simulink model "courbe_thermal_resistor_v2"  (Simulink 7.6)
settings: Solver=ode15s  StartTime=0.0  StopTime=500  RelTol=1e-3
InitFcn:
  | Vcc=12;
  | R=1e3;
  | 
  | T0=25+273.15;
  | R0=1;
  | alpha=5e-5;
StopFcn:
  | close all
  | load Te_appliquee_Tcalculee.mat
  | plot(x(1,:),x(2,:))
  | hold on
  | plot (x(1,:),x(3,:))
  | title('Température appliquée et mesurée')
  | xlabel('temps')
  | grid
undefined symbols (not defined in the file or in its folder): sigbuilder_block
libraries: fl_lib x17, nesl_utility x3, elec_lib x2

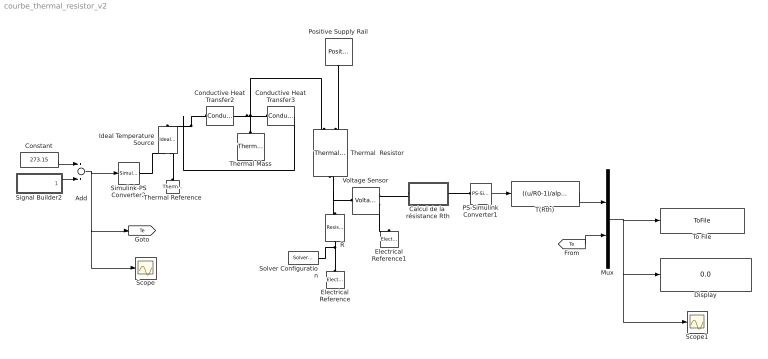
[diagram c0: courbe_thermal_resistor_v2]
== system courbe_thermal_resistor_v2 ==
  Add : Sum  Inputs=2
  Calcul de la  résistance Rth : Subsystem
  Conductive Heat Transfer2 : fl_lib/Thermal/Thermal Elements/Conductive Heat Transfer  DialogController=NetworkEngine.DynNeDlgSource  SystemSampleTime=-1  area=0.04 m^2  thickness=0.1 m  th_cond=46 W/(m*K)  Q_Log=off  T_Log=off  LocalVarNames=|Q|T  LocalVarDescs=|Q|T  LocalVarLogging=[0 0]
  Conductive Heat Transfer3 : fl_lib/Thermal/Thermal Elements/Conductive Heat Transfer  DialogController=NetworkEngine.DynNeDlgSource  SystemSampleTime=-1  area=0.04 m^2  thickness=0.1 m  th_cond=46 W/(m*K)  Q_Log=off  T_Log=off  LocalVarNames=|Q|T  LocalVarDescs=|Q|T  LocalVarLogging=[0 0]
  Constant : Constant  Value=273.15
  Display : Display
  Electrical Reference : fl_lib/Electrical/Electrical Elements/Electrical Reference  DialogController=NetworkEngine.DynNeDlgSource  SystemSampleTime=-1  i_Log=off  LocalVarNames=|i  LocalVarDescs=|i  LocalVarLogging=[]
  Electrical Reference1 : fl_lib/Electrical/Electrical Elements/Electrical Reference  DialogController=NetworkEngine.DynNeDlgSource  SystemSampleTime=-1  i_Log=off  LocalVarNames=|i  LocalVarDescs=|i  LocalVarLogging=[]
  Ideal Temperature Source : fl_lib/Thermal/Thermal Sources/Ideal Temperature Source  DialogController=NetworkEngine.DynNeDlgSource  SystemSampleTime=-1  Q_Log=off  T_Log=off  LocalVarNames=|Q|T  LocalVarDescs=|Q|T  LocalVarLogging=[0 0]
  Mux : Mux  Inputs=2
  PS-Simulink Converter1 : nesl_utility/PS-Simulink Converter  DialogController=NetworkEngine.DynNeUtilDlgSource  SystemSampleTime=-1  PhysicalDomain=network_engine_domain  LeftPortType=input  RightPortType=output  SubClassName=ps_output  Unit=V  AffineConversion=off
  Positive Supply Rail : elec_lib/Sources/Positive Supply Rail  DialogController=NetworkEngine.DynNeDlgSource  SystemSampleTime=-1  v0=Vcc V  current_Log=off  voltage_Log=off  power_Log=off  LocalVarNames=|current|voltage|power  LocalVarDescs=|Current (A)|Voltage (V)|Power (W)  LocalVarLogging=[0 0 0]
  R : fl_lib/Electrical/Electrical Elements/Resistor  DialogController=NetworkEngine.DynNeDlgSource  SystemSampleTime=-1  R=R Ohm  i_Log=off  v_Log=off  LocalVarNames=|current|voltage|power  LocalVarDescs=|Resistor current (A)|Voltage across resistor (V)|Power (W)  LocalVarLogging=[0 0 0]
  Scope : Scope
  Scope1 : Scope
  Signal Builder2 : Subsystem  Tag=STV Subsys  LoadFcn=sigbuilder_block('load');  StartFcn=sigbuilder_block('start');  StopFcn=sigbuilder_block('stop');  ClipboardFcn=sigbuilder_block('clipboard');
  Simulink-PS Converter2 : nesl_utility/Simulink-PS Converter  DialogController=NetworkEngine.DynNeUtilDlgSource  SystemSampleTime=-1  PhysicalDomain=network_engine_domain  LeftPortType=input  RightPortType=output  SubClassName=ps_input  Unit=1  AffineConversion=off  InputFilterTimeConstant=.001  UdotUserProvided=0
  Solver Configuration : nesl_utility/Solver Configuration  DialogController=NetworkEngine.DynNeUtilDlgSource  SystemSampleTime=-1  PhysicalDomain=network_engine_domain  LeftPortType=input  RightPortType=generic  SubClassName=solver  Accelerate=off  Profile=off  ResidualTolerance=1e-9  MaxNonlinIter=12  MaxModeIter=2  DoFixedCost=off  UseLocalSampling=off  DoDC=off  LinearAlgebra=Sparse  LocalSolverSampleTime=.001  LocalSolverChoice=NE_BACKWARD_EULER_ADVANCER  UseLocalSolver=off
  T(Rth) : Fcn  Expr=((u/R0-1)/alpha)+T0
  Thermal Mass : fl_lib/Thermal/Thermal Elements/Thermal Mass  DialogController=NetworkEngine.DynNeDlgSource  SystemSampleTime=-1  mass=1 kg  sp_heat=444 J/kg/K  init_temp=25 C  Q_Log=off  LocalVarNames=|heat_flow|temperature  LocalVarDescs=|Heat flow (J/s)|Mass temperature (K)  LocalVarLogging=[0 0]
  Thermal  Resistor : elec_lib/Passive Devices/Thermal Resistor  DialogController=NetworkEngine.DynNeDlgSource  SystemSampleTime=-1  R0=1 Ohm  T0=25 C  alpha=5e-05 1/K  tc=10 s  K_d=0.001 W/K  init_temp=25 C  current_Log=off  voltage_Log=off  power_Log=off  temperature_Log=off  heat_flow_Log=off  LocalVarNames=|current|voltage|power|temperature|heat_flow  LocalVarDescs=|Resistor current (A)|Voltage across resistor (V)|Power (W)|Themistor temperature (K)|Heat flow (J/s)  LocalVarLogging=[0 0 0 0 0]
  Thermal Reference : fl_lib/Thermal/Thermal Elements/Thermal Reference  DialogController=NetworkEngine.DynNeDlgSource  SystemSampleTime=-1  Q_Log=off  LocalVarNames=|Q  LocalVarDescs=|Q  LocalVarLogging=0
  To File : ToFile  Filename=Te_appliquee_Tcalculee  MatrixName=x
  Voltage Sensor : fl_lib/Electrical/Electrical Sensors/Voltage Sensor  DialogController=NetworkEngine.DynNeDlgSource  SystemSampleTime=-1  i1_Log=off  v1_Log=off  LocalVarNames=|i1|v1  LocalVarDescs=|i1|v1  LocalVarLogging=[]
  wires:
  Mux/1 -> To File/1, Scope1/1, Display/1
  PS-Simulink Converter1/1 -> T(Rth)/1
  T(Rth)/1 -> Mux/1
  [Te] -> Mux/2
  Add/1 -> Simulink-PS Converter2/1, [Te], Scope/1
  Constant/1 -> Add/1
  Signal Builder2/1(Signal 2) -> Add/2
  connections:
  Positive Supply Rail/RConn1 -- Thermal  Resistor/LConn2
  Thermal  Resistor/RConn1 -- R/RConn1 -- Voltage Sensor/LConn1
  Voltage Sensor/RConn2 -- Electrical Reference1/LConn1
  Thermal Reference/LConn1 -- Ideal Temperature Source/RConn2
  Simulink-PS Converter2/RConn1 -- Ideal Temperature Source/RConn1
  Calcul de la  résistance Rth/RConn1 -- PS-Simulink Converter1/LConn1
  Calcul de la  résistance Rth/LConn1 -- Voltage Sensor/RConn1
  R/LConn1 -- Electrical Reference/LConn1 -- Solver Configuration/RConn1
  Ideal Temperature Source/LConn1 -- Conductive Heat Transfer2/LConn1 -- Conductive Heat Transfer3/RConn1
  Conductive Heat Transfer2/RConn1 -- Conductive Heat Transfer3/LConn1 -- Thermal  Resistor/LConn1 -- Thermal Mass/LConn1

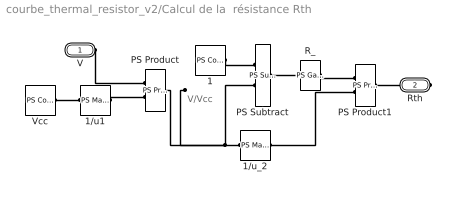
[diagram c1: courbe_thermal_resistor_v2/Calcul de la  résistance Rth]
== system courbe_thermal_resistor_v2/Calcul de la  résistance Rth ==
  note: V/Vcc
  1 : fl_lib/Physical Signals/Sources/PS Constant  DialogController=NetworkEngine.DynNeDlgSource  SystemSampleTime=-1  constant=1  LocalVarLogging=[]
  1/u1 : fl_lib/Physical Signals/Functions/PS Math Function  DialogController=NetworkEngine.DynNeDlgSource  SystemSampleTime=-1  fcn_choice=9  LocalVarLogging=[]
  1/u_2 : fl_lib/Physical Signals/Functions/PS Math Function  DialogController=NetworkEngine.DynNeDlgSource  SystemSampleTime=-1  fcn_choice=9  LocalVarLogging=[]
  PS Product : fl_lib/Physical Signals/Functions/PS Product  DialogController=NetworkEngine.DynNeDlgSource  SystemSampleTime=-1  LocalVarLogging=[]
  PS Product1 : fl_lib/Physical Signals/Functions/PS Product  DialogController=NetworkEngine.DynNeDlgSource  SystemSampleTime=-1  LocalVarLogging=[]
  PS Subtract : fl_lib/Physical Signals/Functions/PS Subtract  DialogController=NetworkEngine.DynNeDlgSource  SystemSampleTime=-1  LocalVarLogging=[]
  R_ : fl_lib/Physical Signals/Functions/PS Gain  DialogController=NetworkEngine.DynNeDlgSource  SystemSampleTime=-1  gain=R  LocalVarLogging=[]
  Vcc : fl_lib/Physical Signals/Sources/PS Constant  DialogController=NetworkEngine.DynNeDlgSource  SystemSampleTime=-1  constant=Vcc  LocalVarLogging=[]
  V : PMIOPort  Port=1  Side=Left
  Rth : PMIOPort  Port=2  Side=Right
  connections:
  1/RConn1 -- PS Subtract/LConn1
  Vcc/RConn1 -- 1/u1/LConn1
  1/u1/RConn1 -- PS Product/LConn2
  1/u_2/LConn1 -- PS Subtract/LConn2 -- PS Product/RConn1
  1/u_2/RConn1 -- PS Product1/LConn2
  R_/RConn1 -- PS Product1/LConn1
  PS Subtract/RConn1 -- R_/LConn1
  V/RConn1 -- PS Product/LConn1
  Rth/RConn1 -- PS Product1/RConn1

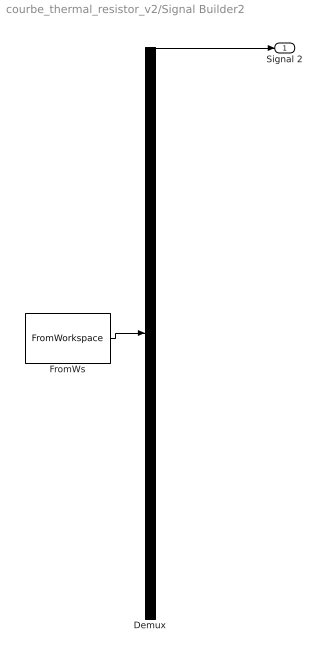
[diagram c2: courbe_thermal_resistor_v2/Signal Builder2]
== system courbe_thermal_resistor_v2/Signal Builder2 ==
  Demux : Demux  Tag=STV Demux  Outputs=1
  FromWs : FromWorkspace  Tag=STV FromWs  VariableName=tuvar  SampleTime=0  SigBuilderData=DataTag0  VnvData=DataTag1
  Signal 2 : Outport  Tag=STV Outport
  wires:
  FromWs/1 -> Demux/1
  Demux/1 -> Signal 2/1
